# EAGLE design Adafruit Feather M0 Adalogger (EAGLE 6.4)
COMPANY: ADAFRUIT INDUSTRIES; DRAWN: KTOWN; REV: B
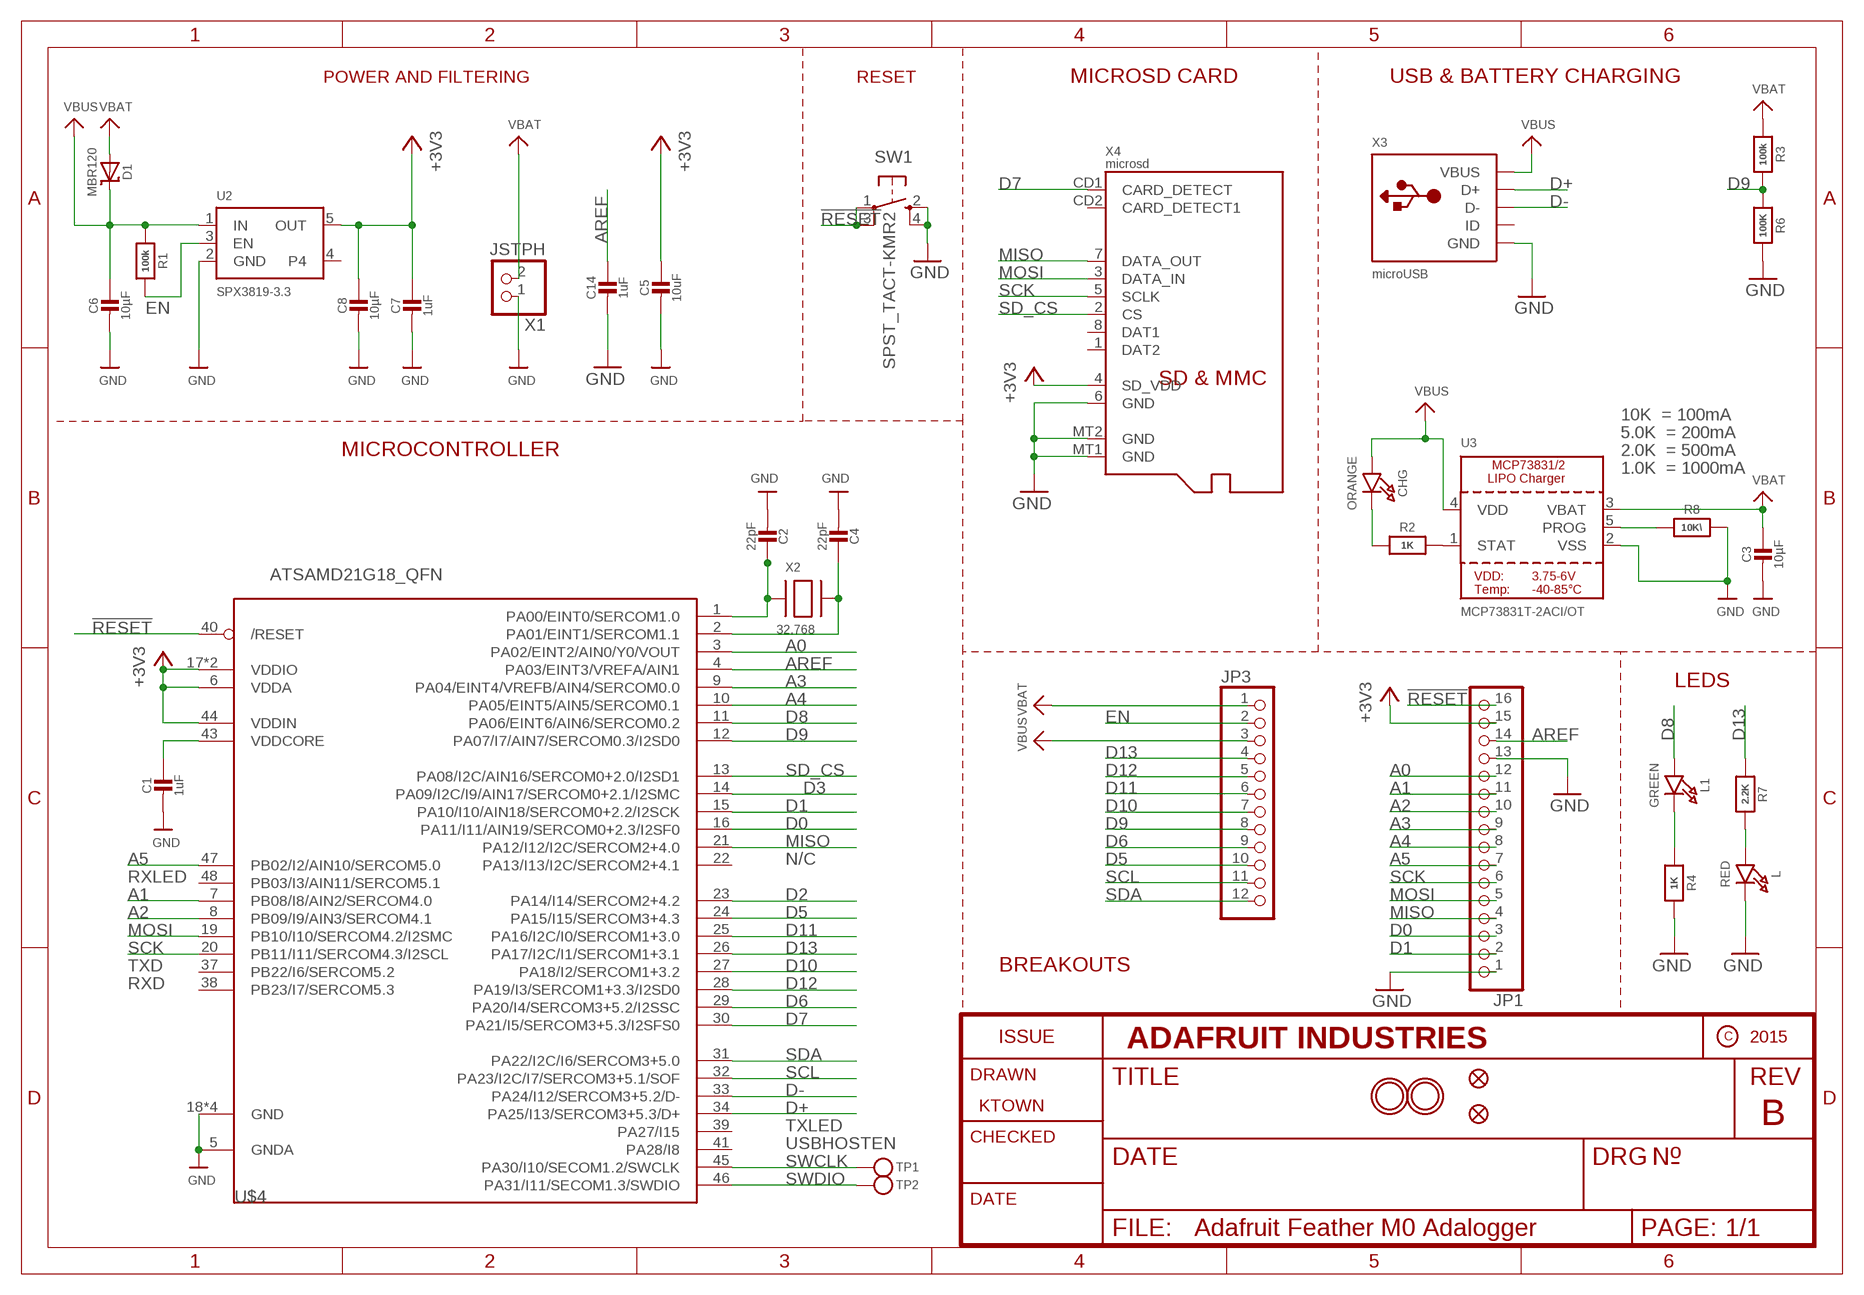
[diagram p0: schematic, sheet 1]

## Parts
C1  1uF  CAP_CERAMIC0603_NO  [0603-NO]
C2  22pF  CAP_CERAMIC0603_NO  [0603-NO]
C3  10µF  CAP_CERAMIC0805-NOOUTLINE  [0805-NO]
C4  22pF  CAP_CERAMIC0603_NO  [0603-NO]
C5  10uF  CAP_CERAMIC0805-NOOUTLINE  [0805-NO]
C6  10µF  CAP_CERAMIC0805-NOOUTLINE  [0805-NO]
C7  1uF  CAP_CERAMIC0603_NO  [0603-NO]
C8  10µF  CAP_CERAMIC0805-NOOUTLINE  [0805-NO]
C14  1uF  CAP_CERAMIC0603_NO  [0603-NO]
CHG  ORANGE  LED0805_NOOUTLINE  [CHIPLED_0805_NOOUTLINE]
D1  MBR120  DIODE-SCHOTTKYSOD-123  [SOD-123]
JP1  HEADER-1X16ROUND  [1X16_ROUND]
JP3  HEADER-1X12  [1X12_ROUND]
L  RED  LED0805_NOOUTLINE  [CHIPLED_0805_NOOUTLINE]
L1  GREEN  LED0805_NOOUTLINE  [CHIPLED_0805_NOOUTLINE]
R1  100k  RESISTOR_0603_NOOUT  [0603-NO]
R2  1K  RESISTOR_0603_NOOUT  [0603-NO]
R3  100k  RESISTOR_0603_NOOUT  [0603-NO]
R4  1K  RESISTOR_0603_NOOUT  [0603-NO]
R6  100K  RESISTOR_0603_NOOUT  [0603-NO]
R7  2.2K  RESISTOR_0603_NOOUT  [0603-NO]
R8  10K\  RESISTOR_0603_NOOUT  [0603-NO]
SW1  SPST_TACT-KMR2  [KMR2]
TP1  TESTPOINTROUND1.5MM  [TESTPOINT_ROUND_1.5MM]
TP2  TESTPOINTROUND1.5MM  [TESTPOINT_ROUND_1.5MM]
U2  SPX3819-3.3  VREG_SOT23-5  [SOT23-5]
U3  MCP73831T-2ACI/OT  MCP73831/2  [SOT23-5]
U$4  ATSAMD21G18_QFN  ATSAMD21J_QFN  [TQFN48_7MM]
U$31  MOUNTINGHOLE2.5  [MOUNTINGHOLE_2.5_PLATED]
U$32  MOUNTINGHOLE2.5  [MOUNTINGHOLE_2.5_PLATED]
U$34  FIDUCIAL""  [FIDUCIAL_1MM]
U$35  FIDUCIAL""  [FIDUCIAL_1MM]
X1  JSTPH  CON_JST_PH_2PIN  [JSTPH2]
X2  32.768  XTAL-3.2X1.5  [XTAL3215]
X3  microUSB  USB_MICRO_20329_V2  [4UCONN_20329_V2]
X4  microsd  MICROSD  [MICROSD]

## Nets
!RESET: JP1.16 SW1.1(P) SW1.3(P1) U$4.40(/RESET)
+3V3: C5.1 C7.1 C8.1 JP1.15 U2.5(OUT) U$4.6(VDDA) U$4.17(VDDIO) U$4.36(VDDIO) U$4.44(VDDIN) X4.4(SD_VDD)
A0: JP1.12 U$4.3(PA02/EINT2/AIN0/Y0/VOUT)
A1: JP1.11 U$4.7(PB08/I8/AIN2/SERCOM4.0)
A2: JP1.10 U$4.8(PB09/I9/AIN3/SERCOM4.1)
A3: JP1.9 U$4.9(PA04/EINT4/VREFB/AIN4/SERCOM0.0)
A4: JP1.8 U$4.10(PA05/EINT5/AIN5/SERCOM0.1)
A5: JP1.7 U$4.47(PB02/I2/AIN10/SERCOM5.0)
AREF: C14.1 JP1.14 U$4.4(PA03/EINT3/VREFA/AIN1)
D0: JP1.3 U$4.16(PA11/I11/AIN19/SERCOM0+2.3/I2SF0)
D1: JP1.2 U$4.15(PA10/I10/AIN18/SERCOM0+2.2/I2SCK)
D2: U$4.23(PA14/I14/SERCOM2+4.2)
D3: U$4.14(PA09/I2C/I9/AIN17/SERCOM0+2.1/I2SMC)
D5: JP3.10 U$4.24(PA15/I15/SERCOM3+4.3)
D6: JP3.9 U$4.29(PA20/I4/SERCOM3+5.2/I2SSC)
D7: U$4.30(PA21/I5/SERCOM3+5.3/I2SFS0) X4.CD1(CARD_DETECT)
D8: L1.A U$4.11(PA06/EINT6/AIN6/SERCOM0.2)
D9: JP3.8 R3.2 R6.1 U$4.12(PA07/I7/AIN7/SERCOM0.3/I2SD0)
D10: JP3.7 U$4.27(PA18/I2/SERCOM1+3.2)
D11: JP3.6 U$4.25(PA16/I2C/I0/SERCOM1+3.0)
D12: JP3.5 U$4.28(PA19/I3/SERCOM1+3.3/I2SD0)
D13: JP3.4 R7.1 U$4.26(PA17/I2C/I1/SERCOM1+3.1)
D+: U$4.34(PA25/I13/SERCOM3+5.3/D+) X3.D+
D-: U$4.33(PA24/I12/SERCOM3+5.2/D-) X3.D-
EN: JP3.2 R1.2 U2.3(EN)
GND: C1.2 C2.2 C3.2 C4.2 C5.2 C6.2 C7.2 C8.2 C14.2 JP1.1 JP1.13 L.C R4.2 R6.2 R8.2 SW1.2(S) SW1.4(S1) U2.2(GND) U3.2(VSS) U$4.5(GNDA) U$4.18(GND) U$4.35(GND) U$4.42(GND) U$4.THERMAL(GND) X1.1 X3.BASE@1(GND) X3.BASE@2(GND) X3.GND X3.SPRT@1(GND) X3.SPRT@2(GND) X3.SPRT@3(GND) X3.SPRT@4(GND) X4.6(GND) X4.MT1(GND) X4.MT2(GND)
MISO: JP1.4 U$4.21(PA12/I12/I2C/SERCOM2+4.0) X4.7(DATA_OUT)
MOSI: JP1.5 U$4.19(PB10/I10/SERCOM4.2/I2SMC) X4.3(DATA_IN)
N$1: CHG.C R2.1
N$2: L.A R7.2
N$3: R2.2 U3.1(STAT)
N$4: R8.1 U3.5(PROG)
N$5: C2.1 U$4.1(PA00/EINT0/SERCOM1.0) X2.P$1
N$6: L1.C R4.1
N$7: C4.1 U$4.2(PA01/EINT1/SERCOM1.1) X2.P$2
SCK: JP1.6 U$4.20(PB11/I11/SERCOM4.3/I2SCL) X4.5(SCLK)
SCL: JP3.11 U$4.32(PA23/I2C/I7/SERCOM3+5.1/SOF)
SD_CS: U$4.13(PA08/I2C/AIN16/SERCOM0+2.0/I2SD1) X4.2(CS)
SDA: JP3.12 U$4.31(PA22/I2C/I6/SERCOM3+5.0)
SWCLK: TP1.P$1 U$4.45(PA30/I10/SECOM1.2/SWCLK)
SWDIO: TP2.P$1 U$4.46(PA31/I11/SECOM1.3/SWDIO)
VBAT: C3.1 D1.A JP3.1 R3.1 U3.3(VBAT) X1.2
VBUS: C6.1 CHG.A D1.C JP3.3 R1.1 U2.1(IN) U3.4(VDD) X3.VBUS
VDDCORE: C1.1 U$4.43(VDDCORE)
Unconnected: U2.4 U$4.22(PA13/I13/I2C/SERCOM2+4.1) U$4.37(PB22/I6/SERCOM5.2) U$4.38(PB23/I7/SERCOM5.3) U$4.39(PA27/I15) U$4.41(PA28/I8) U$4.48(PB03/I3/AIN11/SERCOM5.1) X3.ID X4.1(DAT2) X4.8(DAT1) X4.CD2(CARD_DETECT1)

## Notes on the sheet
- POWER AND FILTERING | RESET | MICROSD CARD | USB & BATTERY CHARGING
- 10K  = 100mA
- 5.0K  = 200mA
- MICROCONTROLLER | 2.0K  = 500mA
- 1.0K  = 1000mA
- LEDS
- N/C
- RXLED
- TXD | BREAKOUTS
- RXD
- TXLED
- USBHOSTEN

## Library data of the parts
C1-C8 C14 = microbuilder:CAP_CERAMIC: Ceramic Capacitors
CHG L L1 = microbuilder:LED: LED
D1 = microbuilder:DIODE-SCHOTTKY
JP1 = microbuilder:HEADER-1X16: PIN HEADER
JP3 = microbuilder:HEADER-1X12
R1-R4 R6-R8 = microbuilder:RESISTOR: Resistors
SW1 = adafruit:SPST_TACT: SMT 6mm switch, EVQQ2 series http://www.ladyada.net/library/eagle
TP1 TP2 = microbuilder:TESTPOINT: Test Point
U2 = microbuilder:VREG_SOT23-5: SOT23-5 Fixed Voltage Regulators Part Current Out V Out V In V Dropout θJA (°C/W) TJ (°C) Digikey Part No. ADP121 150mA 3.3V 3.4-5.5V 0.09V @ 150mA -- -- ADP121-AUJZ33R7CT-ND ADP121 150mA 3.0V 3.1-5.5V 0.09V @ 150mA -- -- ADP121-AUJZ30R7CT-ND ADP122 300mA 3.3V 3.4-5.5V 0.085V @ 300mA -- --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
U3 = microbuilder:MCP73831/2: MCP73831/2 LIPO Charger VDD: 3.75 - 6V Temp -40 - 85°C Programmable Charge Rate: 15-500mA NOTE: STAT is a tri-state logic output on the MCP73831 and an open-drain output on the MCP73832. SOT23-5 with 4.2V output and tri-state logic on STAT = MCP73831T-2ACI/OT
U$4 = microbuilder:ATSAMD21J
U$31 U$32 = microbuilder:MOUNTINGHOLE: Mounting Hole; BOM: EXCLUDE
U$34 U$35 = microbuilder:FIDUCIAL: Fiducial Alignment Points; BOM: EXCLUDE
X1 = microbuilder:CON_JST_PH_2PIN: JST 2-Pin Right-Angle Connector
X2 = adafruit2:XTAL: Low cost SMT crystals, no capacitors included
X3 = microbuilder:USB: USB Connectors USBMINIB - Surface Mount Female Mini-B USB Connector 4UConnector: 06564
X4 = microbuilder:MICROSD: MicroSD/Transflash Card Holder with SPI pinout 3M: 2908-05WB-MG 4UConnector: 19656 Footprint courtesy: Adafruit Industries

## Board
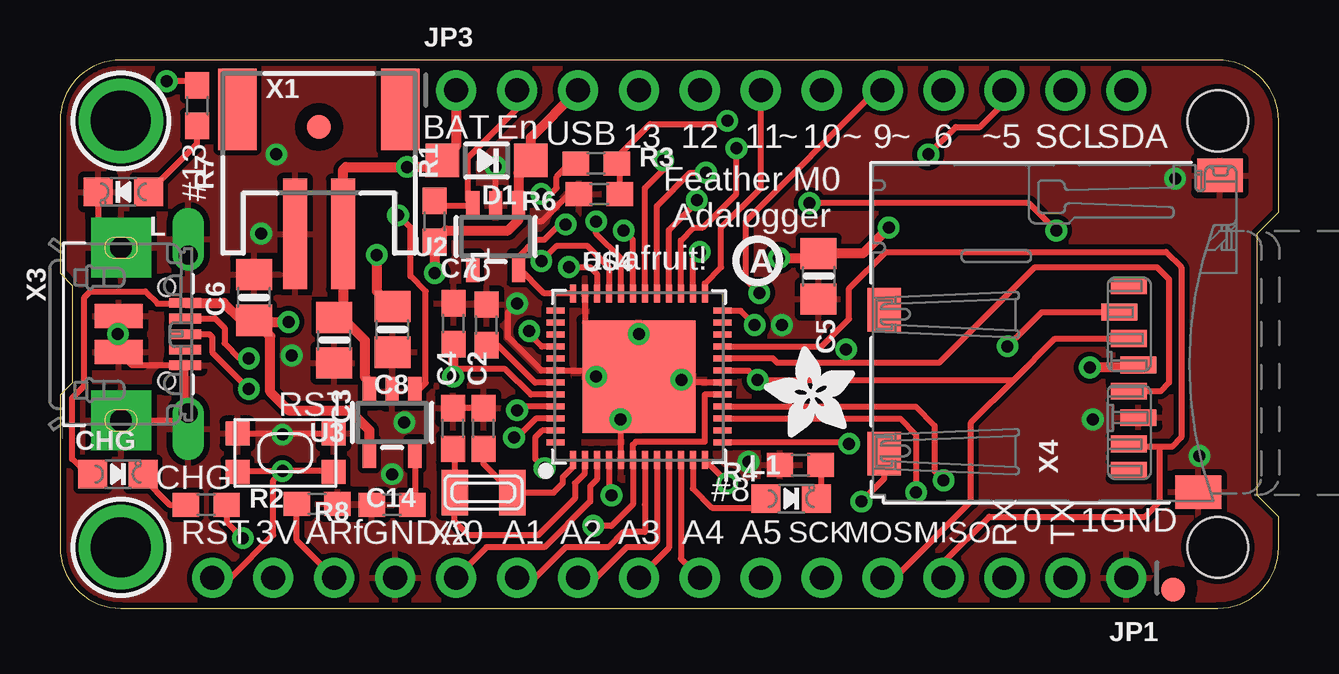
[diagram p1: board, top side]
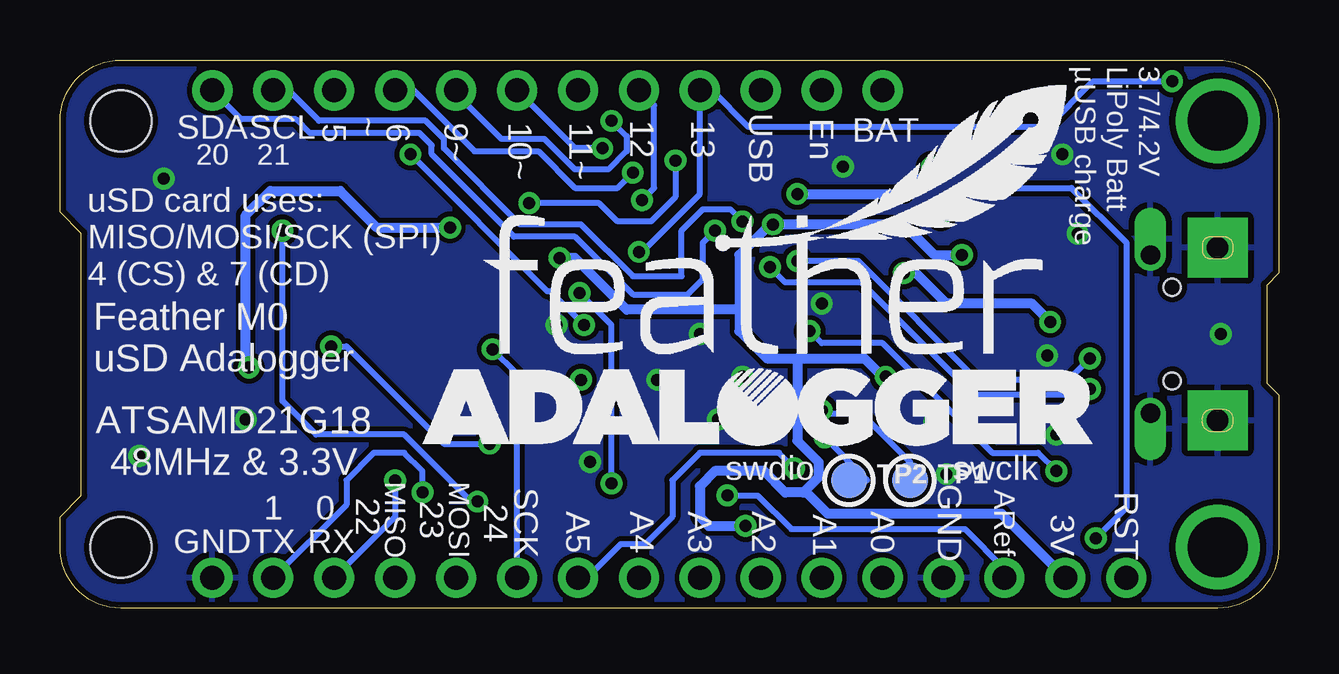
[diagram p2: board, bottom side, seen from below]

Size 50.8 x 22.86 mm. Coordinates in mm from the lower left corner, seen from the top.
Outline: 2.54,0 48.26,0 arc90 50.8,2.54 50.8,3.81 49.91,4.7 49.91,15.62 50.8,16.51 50.8,20.32 arc90 48.26,22.86 2.54,22.86 arc90 0,20.32 0,13.97 0.51,13.46 0.51,9.4 0,8.89 0,2.54 arc90 2.54,0
Copper layers (1*16): Top 0.035mm / dielectric 1.5mm / Bottom 0.035mm
Design rules "adafruit *": minimum track width 8mil, minimum drill 15.5mil, track to track 8mil, track to pad 8mil, pad to pad 8mil, via to via 8mil, smd to smd 8mil, copper to edge 10mil, drill to drill 8mil, minimum pad ring 10mil, minimum via ring 8mil, stop-mask expansion 2mil, vias tented up to drill 20mil, thermal gap 10mil
Holes 2.54 mm at 48.26,20.32 48.26,2.54
tRestrict: area 21.3,6.9 to 21.7,9.7; area 22.1,12.1 to 27.1,12.4; area 26.5,9.7 to 27.1,12.2

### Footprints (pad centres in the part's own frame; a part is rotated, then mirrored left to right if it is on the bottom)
0603-NO = smd 1.1 x 1: 1 -0.85,0; 2 0.85,0
0805-NO = smd 1.3 x 1.5: 1 -0.95,0; 2 0.95,0
CHIPLED_0805_NOOUTLINE = smd 1.2 x 1.2: A 0,-1.05; C 0,1.05
SOD-123 = smd 1.4 x 1.4: A 1.85,0; C -1.85,0
1X16_ROUND = drill 1 pad 1.676: 1 -19.05,0; 2 -16.51,0; 3 -13.97,0; 4 -11.43,0; 5 -8.89,0; 6 -6.35,0; 7 -3.81,0; 8 -1.27,0; 9 1.27,0; 10 3.81,0; 11 6.35,0; 12 8.89,0; 13 11.43,0; 14 13.97,0; 15 16.51,0; 16 19.05,0
1X12_ROUND = drill 1 pad 1.676: 1 -13.97,0; 2 -11.43,0; 3 -8.89,0; 4 -6.35,0; 5 -3.81,0; 6 -1.27,0; 7 1.27,0; 8 3.81,0; 9 6.35,0; 10 8.89,0; 11 11.43,0; 12 13.97,0
KMR2 = smd 1 x 1: 1 2,0.8; 2 2,-0.8; 3 -2,0.8; 4 -2,-0.8
TESTPOINT_ROUND_1.5MM = smd 1.5 x 1.5: P$1 0,0
SOT23-5 = smd 0.55 x 1.2: 1 -0.95,-1.3; 2 0,-1.3; 3 0.95,-1.3; 4 0.95,1.3; 5 -0.95,1.3
TQFN48_7MM = smd 0.25 x 0.75: 1 -2.75,-3.475; 2 -2.25,-3.475; 3 -1.75,-3.475; 4 -1.25,-3.475; 5 -0.75,-3.475; 6 -0.25,-3.475; 7 0.25,-3.475; 8 0.75,-3.475; 9 1.25,-3.475; 10 1.75,-3.475; 11 2.25,-3.475; 12 2.75,-3.475; 25 2.75,3.475; 26 2.25,3.475; 27 1.75,3.475; 28 1.25,3.475; 29 0.75,3.475; 30 0.25,3.475; 31 -0.25,3.475; 32 -0.75,3.475; 33 -1.25,3.475; 34 -1.75,3.475; 35 -2.25,3.475; 36 -2.75,3.475 | smd 0.75 x 0.25: 13 3.475,-2.75; 14 3.475,-2.25; 15 3.475,-1.75; 16 3.475,-1.25; 17 3.475,-0.75; 18 3.475,-0.25; 19 3.475,0.25; 20 3.475,0.75; 21 3.475,1.25; 22 3.475,1.75; 23 3.475,2.25; 24 3.475,2.75; 37 -3.475,2.75; 38 -3.475,2.25; 39 -3.475,1.75; 40 -3.475,1.25; 41 -3.475,0.75; 42 -3.475,0.25; 43 -3.475,-0.25; 44 -3.475,-0.75; 45 -3.475,-1.25; 46 -3.475,-1.75; 47 -3.475,-2.25; 48 -3.475,-2.75 | smd 4.7 x 4.7: THERMAL 0,0
MOUNTINGHOLE_2.5_PLATED = drill 2.5 pad 3.2: P$1 0,0
FIDUCIAL_1MM = smd 1 x 1: 1 0,0
JSTPH2 = smd 1 x 4.6: 1 -1,-3.7; 2 1,-3.7 | smd 1.6 x 3.4: NC1 -3.4,1.5; NC2 3.4,1.5
XTAL3215 = smd 1.1 x 1.9: P$1 1.2,0; P$2 -1.2,0
4UCONN_20329_V2 = smd 1 x 2: BASE@1 -0.75,-2; BASE@2 0.75,-2 | smd 0.4 x 1.35: D+ 0,0.775; D- -0.65,0.775; GND 1.3,0.775; ID 0.65,0.775; VBUS -1.3,0.775 | drill 0.8 pad 1.2 offset: SPRT@1 -3.3,0.9; SPRT@2 3.3,0.9 | drill 0.9 pad 2.5 square: SPRT@3 -3.6,-1.9; SPRT@4 3.6,-1.9 | hole 0.7: -1.95,0; 1.95,0
MICROSD = smd 0.7 x 1.5: 1 9,-10.64; 2 7.9,-10.24; 3 6.8,-10.64; 4 5.7,-11.04; 5 4.6,-10.64; 6 3.5,-11.04; 7 2.4,-10.64; 8 1.3,-10.64 | smd 1.8 x 1.4: CD1 2,-0.44; CD2 8,-0.44 | smd 1.4 x 1.9: MT1 0.4,-13.54; MT2 13.6,-14.44

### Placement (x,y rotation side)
C1  17.78,11.81 90 top
C2  17.65,7.49 90 top
C3  11.43,11.18 270 top
C4  16.38,7.49 90 top
C5  31.62,13.84 270 top
C6  8.09,12.96 90 top
C7  16.4,11.86 90 top
C8  13.86,11.62 270 top
C14  10.72,4.34 0 top
CHG  2.41,5.59 270 top
D1  17.78,18.67 180 top
JP1  25.4,1.27 180 top
JP3  30.48,21.59 0 top
L  2.65,17.36 90 top
L1  30.48,4.57 270 top
R1  15.62,16.13 90 top
R2  6.1,4.32 0 top
R3  22.35,18.54 0 top
R4  30.86,5.97 180 top
R6  22.48,17.27 180 top
R7  5.71,20.95 270 top
R8  13.84,4.32 180 top
SW1  9.4,6.48 180 top
TP1  15.37,5.33 0 bottom
TP2  17.91,5.33 0 bottom
U2  18.16,15.49 180 top
U3  13.84,7.75 180 top
U$4  24.13,9.65 0 top
U$7  [ADAFRUIT_3.5MM]  33.15,7.11 90 top
U$9  [PCBFEAT-REV-040]  29.08,14.48 0 top
U$13  [FEATHERLOGO]  33.15,10.54 0 bottom
U$14  [ADALOGGER_LOGO]  35.69,6.73 0 bottom
U$31  2.54,20.32 270 top
U$32  2.54,2.54 270 top
U$34  10.79,20.07 270 top
U$35  46.4,0.77 270 top
X1  10.79,19.3 0 top
X2  17.65,4.83 0 top
X3  4.45,11.43 270 top
X4  33.91,4.45 90 top

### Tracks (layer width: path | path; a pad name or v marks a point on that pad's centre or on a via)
!RESET  (via drill 0.5)
  Top 0.254: 6.48,1.27 JP1.16 7.11,1.27 8.89,3.05 8.89,5.33 v9.27,5.71 | U$4.40 20.09,10.9 19.56,11.43 v19.56,11.56 | SW1.1 7.44,5.71 v9.27,5.71 | SW1.3 11.36,5.71 v9.27,5.71
  Bottom 0.254: v9.27,5.71 10.03,6.48 11.94,6.48 16.51,11.05 19.05,11.05 v19.56,11.56
+3V3  (via drill 0.5)
  Top 0.254: U$4.44 19.63,8.9 18.56,9.97 16.57,9.97 16.4,10.14 C7.1 | v22.23,3.43 22.99,3.43 23.88,4.32 U$4.6 23.88,6.81 24,6.93 26.87,6.93 26.87,8.9 U$4.17 | 16.4,10.04 C7.1 | U$4.36 20.18,13.13 U2.5 19.11,14.67 19.81,15.37 20.19,15.37 20.83,16 v21.08,16 | 16.38,10.49 16.4,10.5 C7.1
  Top 0.406: v29.97,14.61 31.5,14.61 31.62,14.73 C5.1 33.46,14.79 v34.54,15.88 | v13.21,14.73 13.21,13.22 C8.1 | 16.38,10.49 v16.38,9.65 | X4.4 44.84,10.03 v42.93,10.03
  Bottom 0.254: 21.21,16 v21.08,16
  Bottom 0.406: v22.23,3.43 23.75,3.43 24.13,3.81 24.13,5.08 23.5,5.71 21.46,5.71 20.57,4.83 19.81,4.83 19.68,4.95 | 21.21,16 22.48,14.73 22.48,12.57 | 22.48,12.57 22.48,11.56 21.34,10.41 20.07,10.41 | 20.07,10.41 17.27,10.41 16.38,9.53 v16.38,9.65 | v13.21,14.73 14.35,14.73 15.62,16 v21.08,16 | 22.48,12.57 22.61,12.45 27.18,12.45 29.34,14.61 v29.97,14.61 | 20.07,10.41 20.07,6.99 19.18,6.1 19.18,5.46 19.68,4.95 | JP1.15 11.56,3.94 18.8,3.94 19.68,4.83 19.68,4.95 | v42.93,10.03 43.05,10.16 43.05,16.38 42.04,17.4 39.12,17.4 37.59,15.88 v34.54,15.88
A0
  Top 0.254: U$4.3 22.38,5.36 22.1,5.08 22.1,4.45 20.19,2.54 17.78,2.54 JP1.12
A1
  Top 0.254: U$4.7 24.38,4.31 24.38,3.17 23.5,3.17 22.86,2.54 21.08,2.54 19.81,1.27 JP1.11
A2
  Top 0.254: U$4.8 24.88,2.78 24.64,2.54 23.62,2.54 22.35,1.27 JP1.10 21.84,1.27
A3
  Top 0.254: U$4.9 25.38,2.52 JP1.9
A4
  Top 0.254: U$4.10 25.88,2.06 JP1.8
A5  (via drill 0.5)
  Top 0.254: U$4.47 20.1,7.4 19.81,7.11 19.81,6.22 v20.19,5.84
  Bottom 0.254: v20.19,5.84 20.83,6.48 24.13,6.48 25.27,5.33 25.27,3.81 26.42,2.67 27.43,2.67 28.83,1.27 JP1.7
AREF  (via drill 0.5)
  Top 0.254: JP1.14 9.87,2.83 C14.1 | U$4.4 22.88,4.81 v22.99,4.7
  Bottom 0.254: 11.43,1.78 JP1.14 11.43,1.65 13.08,3.3 20.32,3.3 21.72,4.7 v22.99,4.7
D0  (via drill 0.5)
  Top 0.254: U$4.16 35.67,8.4 36.45,7.62 36.45,5.71 v36.83,5.33
  Bottom 0.254: v36.83,5.33 36.83,3.81 JP1.3
D1  (via drill 0.5)
  Top 0.254: U$4.15 35.02,7.9 35.69,7.24 v35.69,4.83
  Bottom 0.254: v35.69,4.83 35.69,5.71 36.45,6.48 37.72,6.48 38.86,5.33 38.86,4.32 JP1.2
D5  (via drill 0.5)
  Top 0.254: U$4.24 28.36,12.4 v28.96,11.81 | v36.2,18.92 37.34,20.07 38.35,20.07 39.37,21.08 JP3.10
  Bottom 0.254: v28.96,11.81 30.35,13.21 30.48,13.21 v36.2,18.92
D6  (via drill 0.5)
  Top 0.254: U$4.29 24.88,16.78 26.27,18.16 26.29,18.16 26.42,18.16 v26.92,18.16
  Bottom 0.254: JP3.9 36.07,21.59 33.53,19.05 30.86,19.05 29.34,17.53 27.56,17.53 v26.92,18.16
D7  (via drill 0.5)
  Top 0.254: U$4.30 24.38,17.52 25.15,18.29 v25.15,18.67 | X4.CD1 34.35,5.39 v33.4,4.45 | v41.53,15.75 40.39,16.89 v31.24,16.89
  Bottom 0.254: v25.15,18.67 25.15,17.14 26.16,16.13 27.56,16.13 28.32,16.89 v31.24,16.89 | v33.4,4.45 33.66,4.45 36.45,7.24 40.13,7.24 41.53,8.64 v41.53,15.75
D8
  Top 0.254: U$4.11 26.38,4.99 27.18,4.19 29.05,4.19 L1.A
D9  (via drill 0.5)
  Top 0.254: JP3.8 34.04,21.59 28.57,16.13 28.57,13.72 v29.15,13.14 | U$4.12 27.81,5.24 v27.81,5.21 | v27.81,20.32 27.69,20.19 24.6,20.19 23.2,18.8 R3.2 23.33,18.41 R6.1
  Bottom 0.254: v29.15,13.14 27.81,11.81 v27.81,5.21 | v27.81,20.32 27.18,19.68 27.18,19.05 27.94,18.29 29.34,18.29 30.61,19.56 32.38,19.56 34.29,21.46 JP3.8
D10  (via drill 0.5)
  Top 0.254: U$4.27 25.88,15.34 26.42,15.88 26.8,15.88 28.19,17.27 v28.19,19.18
  Bottom 0.254: 31.62,21.46 JP3.7 29.34,19.18 v28.19,19.18
D11
  Top 0.254: U$4.25 26.88,13.54 27.56,14.22 27.56,15.88 29.21,17.53 JP3.6
D12  (via drill 0.5)
  Top 0.254: U$4.28 25.38,15.77 26.54,16.93 v26.54,17.02
  Bottom 0.254: v26.54,17.02 26.04,17.53 26.04,20.95 JP3.5
D13  (via drill 0.5)
  Top 0.254: U$4.26 26.38,14.57 v26.67,14.86 | R7.1 5.55,21.97 v4.45,21.97
  Bottom 0.254: v4.45,21.97 7.75,21.97 9.65,20.07 22.1,20.07 23.62,21.59 JP3.4 24.13,17.27 26.67,14.73 v26.67,14.86
D+  (via drill 0.5)
  Top 0.254: X3.D+ 6.22,11.43 6.35,11.3 6.35,10.67 v7.87,9.14 | v21.21,14.22 22.1,14.22 22.38,13.94 U$4.34
  Bottom 0.254: v7.87,9.14 8.13,8.89 12.7,8.89 17.4,13.59 20.57,13.59 v21.21,14.22
D-  (via drill 0.5)
  Top 0.254: X3.D- 6.46,12.08 6.86,11.68 6.86,11.05 7.49,10.41 v7.87,10.41 | v20.07,14.48 20.7,15.11 21.97,15.11 22.88,14.2 U$4.33
  Bottom 0.254: v7.87,10.41 8.76,9.53 12.57,9.53 17.53,14.48 v20.07,14.48
EN
  Top 0.254: JP3.2 19.05,20.83 17.02,18.8 17.02,16.99 U2.3 15.81,16.79 R1.2
GND  (via drill 0.5)
  Top 0.254: L.C 1.59,15.03 X3.SPRT@3 | X3.BASE@2 3,10.13 X3.GND 5.22,8.26 X3.SPRT@2 5.04,7.83 X3.SPRT@4 | SW1.2 SW1.4 11.52,7.28 | 13.97,10.67 C8.2 | U$4.35 21.88,11.9 U$4.THERMAL | U$4.THERMAL 23.88,9.9 U$4.42 20.07,9.9 18.67,11.3 18.67,12.32 v19.05,12.7 | U$4.5 23.38,8.9 | 23.38,8.9 U$4.THERMAL | U$4.18 24.38,9.4 U$4.THERMAL | C2.2 C4.2 | U2.2 18.16,18.03 | 19.94,16.13 20.07,16.13 21.34,17.4 21.46,17.27 R6.2 | 23.38,8.9 23.37,8.89 v23.37,7.87
  Bottom 0.254: v28.7,6.1 28.57,5.97
  other vias: 2.41,11.43 9.65,10.54 9.02,18.92 13.84,5.59 9.27,7.24 18.16,18.41 22.35,9.65 24.13,11.43 25.91,9.53 14.35,7.75 8.38,15.62 43.05,7.87 47.5,6.35 46.48,17.91 30.1,11.81
  pour Top: 0,22.86 0,0 50.93,-0.13 50.93,22.73
  pour Bottom: 50.93,0 0,0 0,22.86 50.93,22.86
MISO
  Top 0.254: U$4.21 31.73,10.9 32.89,12.06 32.89,13.34 34.42,14.86 46.1,14.86 46.74,14.22 46.74,7.11 46.35,6.73 45.85,6.73 | JP1.4 36.83,1.91 38.73,3.81 45.21,3.81 45.85,4.45 45.85,6.73 | 45.85,6.73 44.66,6.73 X4.7
MOSI  (via drill 0.5)
  Top 0.254: U$4.19 28.71,9.9 v29.08,9.53 39.75,9.53 | JP1.5 34.8,1.27 37.97,4.45 37.97,7.75 39.75,9.53 | 39.75,9.53 41.47,11.24 X4.3
N$1
  Top 0.254: CHG.C 3.46,5.43 4.57,4.32 R2.1
N$2
  Top 0.254: L.A 5.71,19.38 R7.2
N$3  (via drill 0.5)
  Top 0.254: U3.1 14.89,9.05 15.24,9.4 15.24,13.21 14.61,13.84 14.61,15.88 v14.1,16.38 | R2.2 6.95,3.6 v7.62,2.92
  Bottom 0.254: v7.62,2.92 6.35,4.19 6.35,15.24 8.64,17.53 13.08,17.53 14.1,16.51 v14.1,16.38
N$4
  Top 0.254: U3.5 14.79,4.42 R8.1
N$5
  Top 0.254: U$4.1 21.38,5.89 20.95,5.46 20.95,5.21 20.57,4.83 X2.P$1 17.65,6.03 C2.1
N$6
  Top 0.254: R4.1 31.71,4.75 L1.C
N$7
  Top 0.254: U$4.2 21.88,5.62 21.46,5.21 21.46,4.57 19.94,3.05 17.02,3.05 16.45,3.61 X2.P$2 16.45,6.57 C4.1
SCK  (via drill 0.5)
  Top 0.254: U$4.20 27.62,10.41 29.72,10.41 29.9,10.24 32.89,10.24 | 32.89,10.24 36.65,10.24 40.64,14.22 45.72,14.22 46.23,13.72 46.23,9.4 45.88,9.04 X4.5 | v32.77,10.79 32.77,10.36 32.89,10.24
  Bottom 0.254: JP1.6 31.75,9.78 v32.77,10.79
SCL  (via drill 0.5)
  Top 0.254: U$4.32 23.38,14.59 22.35,15.62 v22.35,16.13 22.35,16
  Bottom 0.254: JP3.11 41.27,21.59 40.01,20.32 35.56,20.32 34.8,19.56 34.8,19.18 31.62,16 29.08,16 26.92,13.84 24.89,13.84 24.89,15.75 24,16.64 22.86,16.64 v22.35,16.13
SD_CS  (via drill 0.5)
  Top 0.254: v39.5,10.92 40.92,12.35 X4.2 | v32.89,6.86 32.85,6.9 U$4.13
  Bottom 0.254: v39.5,10.92 38.86,10.92 34.8,6.86 v32.89,6.86
SDA  (via drill 0.5)
  Top 0.254: U$4.31 23.88,15.36 v23.5,15.75
  Bottom 0.254: JP3.12 43.24,20.38 40.96,20.38 40.39,19.81 35.81,19.81 35.31,19.3 35.31,18.92 31.88,15.49 29.34,15.49 26.92,13.08 24.64,13.08 24,13.72 24,15.24 v23.5,15.75
SWCLK  (via drill 0.5)
  Top 0.254: U$4.45 19.2,8.4 v19.05,8.26
  Bottom 0.254: v19.05,8.26 18.92,8.13 17.4,8.13 15.37,6.1 TP1.P$1
SWDIO  (via drill 0.5)
  Top 0.254: U$4.46 19.84,7.9 19.05,7.11 v18.92,7.11
  Bottom 0.254: 19.05,7.11 v18.92,7.11 17.14,5.33 TP2.P$1
VBAT  (via drill 0.5)
  Top 0.254: X1.2 11.81,15.62 | 11.79,12.49 C3.1 | v20.07,17.27 20.45,17.27 20.7,17.53 20.7,18 21.25,18.54 R3.1
  Top 0.406: 11.81,15.62 11.81,18.29 11.92,18.4 v14.46,18.4 15.66,18.4 D1.A 16.51,19.25 JP3.1 | X1.2 11.79,12.49 | C3.1 11.75,12.13 12.7,11.18 12.7,9.65 12.89,9.46 U3.3
  Bottom 0.406: v20.07,17.27 15.59,17.27 v14.46,18.4
VBUS  (via drill 0.5)
  Top 0.254: CHG.A 1.14,5.59 0.51,6.22 0.51,8.76 1.02,9.27 1.02,12.95 1.27,13.21 3.56,13.21 4.06,12.7 5.19,12.7 X3.VBUS | 7.55,12.01 C6.1 8.16,11.94
  Top 0.406: X3.VBUS 6.83,12.73 7.55,12.01 | JP3.3 19.63,19.63 D1.C 19.11,18.15 U2.1 19.11,16.19 18.67,15.75 16.09,15.75 R1.1 v15.62,13.97 | U3.4 12.89,7.43 12.06,8.26 9.53,8.26 8.76,9.02 8.76,11.33 C6.1 | 8.16,11.94 v9.53,11.94
  Bottom 0.406: v9.53,11.94 10.29,12.7 13.84,12.7 15.11,13.97 v15.62,13.97
VDDCORE
  Top 0.254: U$4.43 19.81,9.4 18.25,10.96 C1.1

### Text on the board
tPlace: BAT | En | USB | 13 | 12 | 11 | ~ | 10 | ~ | 9 | ~ | 6 | ~5 | SCL | SDA | #13 | Feather M0 / Adalogger | adafruit! | RST | CHG | #8 | RX | 0 | TX | 1 | GND | RST | 3V | ARf | GND | A0 | A1 | A2 | A3 | A4 | A5 | SCK | MOSI | MISO
bPlace: 3.7/4.2V / LiPoly Batt / µUSB charge | BAT | En | 13 | 12 | 6 | ~ | 5 | SCL | SDA | USB | 11~ | 10~ | 9~ | 21 | 20 | uSD card uses: / MISO/MOSI/SCK (SPI) / 4 (CS) & 7 (CD) | Feather M0 / uSD Adalogger | ATSAMD21G18 / 48MHz & 3.3V | swclk | swdio | ARef | GND | SCK | 24 | MOSI | 23 | MISO | 22 | 0 | 1 | RST | 3V | A0 | A1 | A2 | A3 | A4 | A5 | RX | TX | GND

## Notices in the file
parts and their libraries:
microbuilder: This work is placed in the public domain, and may be freely used for commercial and non-commercial work with the following conditions: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
